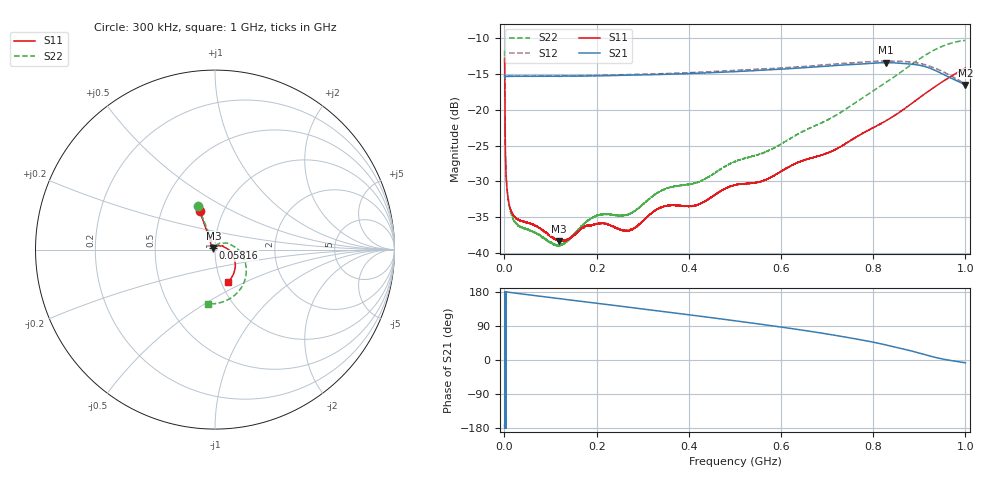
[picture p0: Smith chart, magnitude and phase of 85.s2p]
!Keysight Technologies,N5232A,MY52221221,A.10.65.11
!Date: Thursday, June 15, 2023 18:11:05
!Correction: S11(Full 2 Port(1,4))
!S41(Full 2 Port(1,4))
!S14(Full 2 Port(1,4))
!S44(Full 2 Port(1,4))
!S2P File: Measurements: S11, S41, S14, S44:
# Hz S  RI  R 50
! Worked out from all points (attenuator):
!   16001 points, 300 kHz to 1 GHz, reference 50 ohm
!   highest |S21| = -13.42 dB at 826.8 MHz (marker M1); lowest = -16.6 dB at 999.9 MHz (marker M2)
!   lowest |S11| = -38.3 dB at 117.5 MHz (marker M3), VSWR 1.02, Z = 49.2 + j0.849 ohm
!   |S11| at or under -10 dB: start of sweep to end of sweep
!   |S22| runs from -39.0 to -10.3 dB; largest |S21 - S12| = 0.43
!   S11 on the Smith chart (normalised r, x): 300 kHz: 0.78, +0.35; 58.16 MHz: 0.97, +0.02; 1 GHz: 1.08, -0.41
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300000  -0.0842 0.213  -0.1719 -0.0246  -0.1667 -0.0306  -0.0953 0.2411
6360681  -0.0194 0.0178  -0.1709 0.00163  -0.1716 -0.00311  -0.0175 0.02
1.179655e7  -0.0166 0.0127  -0.1711 0.00462  -0.1716 -0.00402  -0.0142 0.0145
2.62922e7  -0.0144 0.00955  -0.1709 0.0116  -0.1716 -0.0074  -0.0115 0.0112
5.815764e7  -0.0134 0.00877  -0.1693 0.0262  -0.1715 -0.015  -0.01 0.0102
1.174523e8  -0.00847 0.00864  -0.163 0.0524  -0.1693 -0.0325  -0.00529 0.00986
1.408203e8  -0.00609 0.011  -0.1599 0.0628  -0.1685 -0.0378  -0.00293 0.0122
1.669375e8  -0.00488 0.014  -0.1555 0.0734  -0.167 -0.0453  -0.0015 0.0152
2.041763e8  -0.00384 0.0156  -0.1482 0.0885  -0.1651 -0.0552  -0.0019 0.0183
2.690943e8  9.48e-05 0.0143  -0.1324 0.1136  -0.1604 -0.0726  0.00192 0.0185
3.33575e8  0.00579 0.0195  -0.112 0.136  -0.1545 -0.089  0.00833 0.025
4.159878e8  0.00947 0.0193  -0.0811 0.1605  -0.1455 -0.1101  0.0129 0.0281
5.0015e8  0.0186 0.0233  -0.0431 0.1795  -0.1356 -0.1308  0.0258 0.0351
5.585075e8  0.0235 0.0214  -0.013 0.1885  -0.1286 -0.1441  0.034 0.0362
6.667875e8  0.0414 0.0203  0.0514 0.1916  -0.1146 -0.1666  0.0664 0.036
7.187094e8  0.0512 0.014  0.0866 0.1845  -0.1111 -0.1768  0.0872 0.0274
8.26802e8  0.083 -0.00812  0.1636 0.1368  -0.114 -0.1866  0.1519 -0.0289
8.33425e8  0.0851 -0.0109  0.1678 0.1312  -0.1145 -0.1862  0.1557 -0.036
9.227107e8  0.1129 -0.0773  0.1919 0.0362  -0.1223 -0.1597  0.155 -0.1974
9.659477e8  0.1037 -0.1331  0.168 -0.00239  -0.1104 -0.1352  0.0673 -0.2815
9.999375e8  0.0728 -0.1812  0.1475 -0.019  -0.0912 -0.1201  -0.039 -0.3021
1e9  0.0728 -0.1813  0.1475 -0.0192  -0.0913 -0.1199  -0.0392 -0.302
